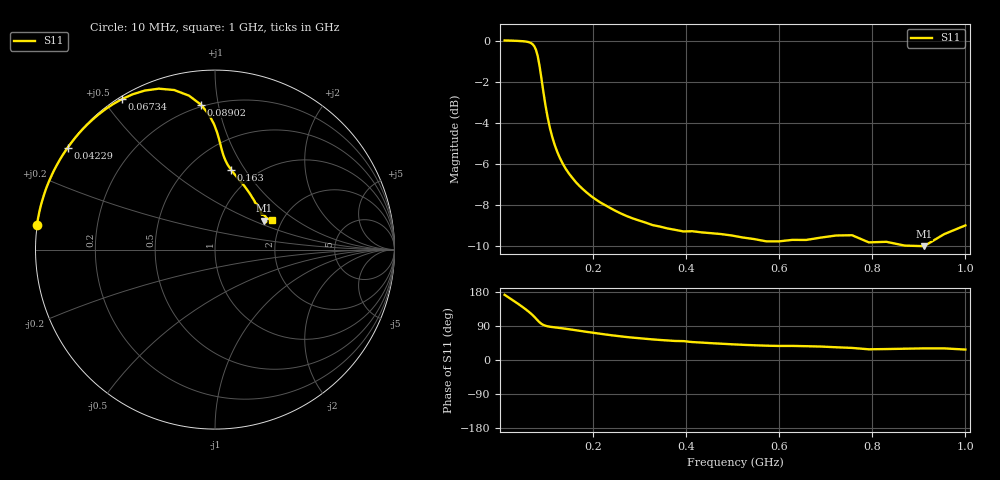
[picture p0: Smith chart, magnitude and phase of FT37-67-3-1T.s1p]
! ListType=Log
!!FT37-67 X 3 1T t2s 12-term
# MHz S RI R 50
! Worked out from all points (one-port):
!   100 points, 10 MHz to 1 GHz, reference 50 ohm
!   lowest |S11| = -10.0 dB at 911.2 MHz (marker M1), VSWR 1.93, Z = 81 + j29.1 ohm
!   |S11| at or under -10 dB: nowhere
!   S11 on the Smith chart (normalised r, x): 10 MHz: -0.00, +0.07; 42.29 MHz: 0.00, +0.31; 67.34 MHz: 0.01, +0.56; 89.02 MHz: 0.19, +0.89; 163 MHz: 0.77, +0.87; 1 GHz: 1.76, +0.66
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10  -0.9915 0.1398
25.35364  -0.9373 0.3498
42.29243  -0.8212 0.5672
55.9081  -0.6808 0.7257
67.34151  -0.5165 0.8396
73.90722  -0.3915 0.8859
77.42637  -0.3136 0.8966
81.11308  -0.2276 0.8891
84.97534  -0.1446 0.8576
89.02151  -0.078 0.8073
93.26033  -0.0328 0.7508
97.701  -0.00493 0.6976
107.2267  0.023 0.6139
117.6812  0.0376 0.5564
135.3048  0.0577 0.4982
162.9751  0.0899 0.4441
205.6512  0.1343 0.3889
259.5024  0.1762 0.3371
327.4549  0.2073 0.29
394.4206  0.2219 0.2627
521.4008  0.2543 0.2141
572.2368  0.2572 0.1992
657.9332  0.2638 0.1947
756.4633  0.2859 0.1778
792.4829  0.2849 0.1531
911.1628  0.2723 0.1616
954.5485  0.2913 0.1729
1000  0.3154 0.1644
